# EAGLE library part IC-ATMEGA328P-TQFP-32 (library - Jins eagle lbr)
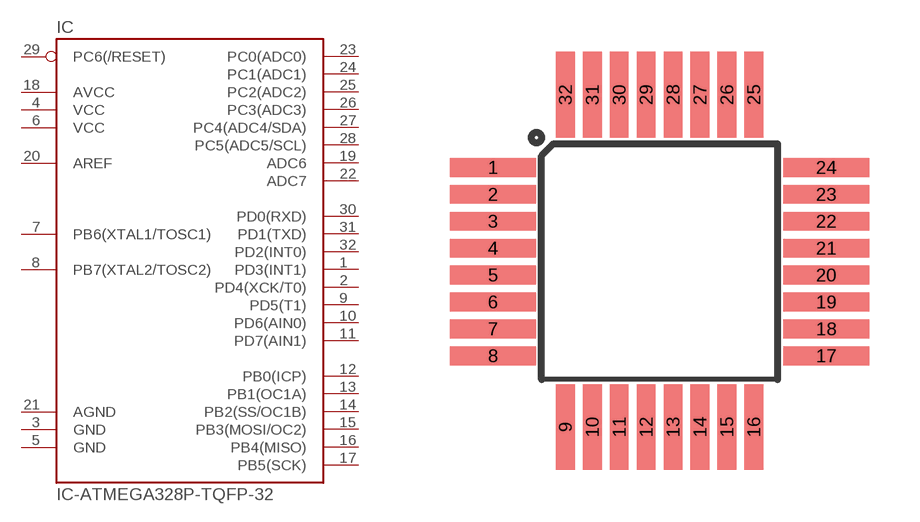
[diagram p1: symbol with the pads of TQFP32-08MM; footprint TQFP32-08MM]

Designator prefix IC

## IC-ATMEGA328P-TQFP-32  [TQFP32-08MM]
1  PD3(INT1)
2  PD4(XCK/T0)
3  GND
4  VCC
5  GND
6  VCC
7  PB6(XTAL1/TOSC1)
8  PB7(XTAL2/TOSC2)
9  PD5(T1)
10  PD6(AIN0)
11  PD7(AIN1)
12  PB0(ICP)
13  PB1(OC1A)
14  PB2(SS/OC1B)
15  PB3(MOSI/OC2)
16  PB4(MISO)
17  PB5(SCK)
18  AVCC
19  ADC6
20  AREF
21  AGND
22  ADC7
23  PC0(ADC0)
24  PC1(ADC1)
25  PC2(ADC2)
26  PC3(ADC3)
27  PC4(ADC4/SDA)
28  PC5(ADC5/SCL)
29  PC6(/RESET)
30  PD0(RXD)
31  PD1(TXD)
32  PD2(INT0)

## Footprint TQFP32-08MM (pad centres in mm)
smd 2.54 x 0.559: 1 -6.502,6.75; 2 -6.502,5.95; 3 -6.502,5.15; 4 -6.502,4.35; 5 -6.502,3.55; 6 -6.502,2.75; 7 -6.502,1.95; 8 -6.502,1.15; 17 3.404,1.15; 18 3.404,1.95; 19 3.404,2.75; 20 3.404,3.55; 21 3.404,4.35; 22 3.404,5.15; 23 3.404,5.95; 24 3.404,6.75
smd 0.559 x 2.54: 9 -4.35,-0.965; 10 -3.55,-0.965; 11 -2.75,-0.965; 12 -1.95,-0.965; 13 -1.15,-0.965; 14 -0.35,-0.965; 15 0.45,-0.965; 16 1.25,-0.965; 25 1.25,8.915; 26 0.45,8.915; 27 -0.35,8.915; 28 -1.15,8.915; 29 -1.95,8.915; 30 -2.75,8.915; 31 -3.55,8.915; 32 -4.35,8.915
